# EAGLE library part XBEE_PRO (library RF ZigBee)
XBee , ZigBee transceiver Producted by XBee ; Digi-Key.Co
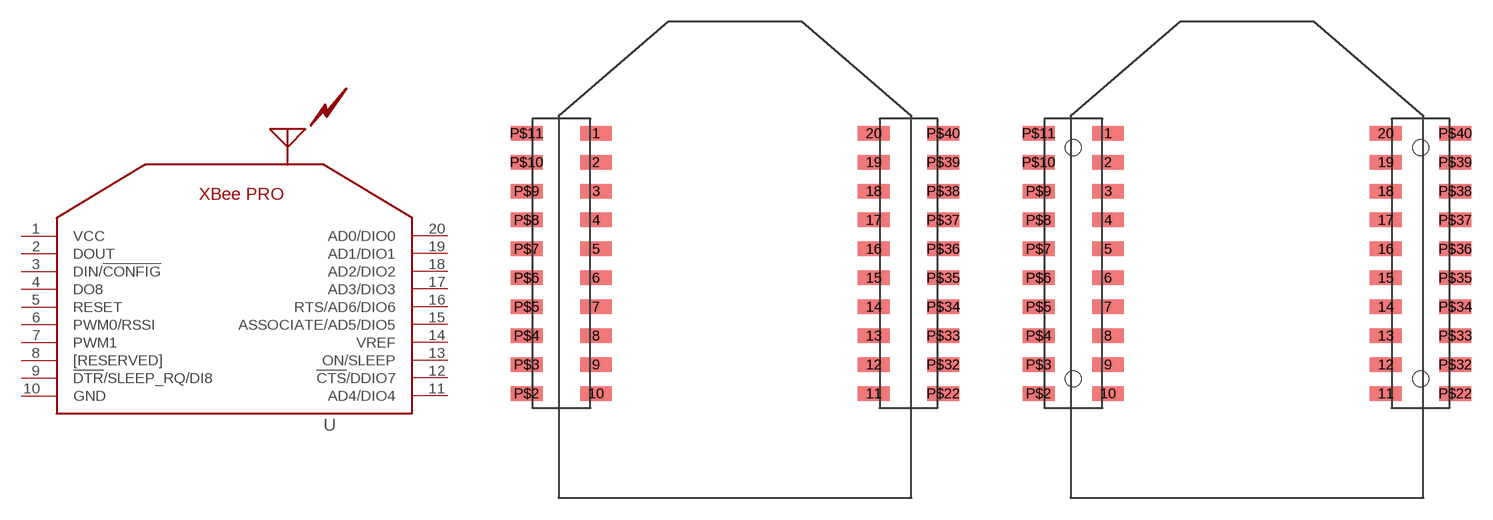
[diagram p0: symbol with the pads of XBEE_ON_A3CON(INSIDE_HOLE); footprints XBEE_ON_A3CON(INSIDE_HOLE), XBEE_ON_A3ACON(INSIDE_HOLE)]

Designator prefix U

## XBEE_PROA3-INSIDE_HOLE  [XBEE_ON_A3CON(INSIDE_HOLE)]
1  VCC
2  DOUT
3  DIN/!CONFIG
4  DO8
5  RESET
6  PWM0/RSSI
7  PWM1
8  [RESERVED]
9  !DTR!/SLEEP_RQ/DI8
10  GND
11  AD4/DIO4
12  !CTS!/DDIO7
13  ON/SLEEP
14  VREF
15  ASSOCIATE/AD5/DIO5
16  RTS/AD6/DIO6
17  AD3/DIO3
18  AD2/DIO2
19  AD1/DIO1
20  AD0/DIO0

## XBEE_PROA3A-INSIDE_HOLE  [XBEE_ON_A3ACON(INSIDE_HOLE)]
Pads as for XBEE_ON_A3CON(INSIDE_HOLE)

## XBEE_PRONPPN101BFLD-RC  [XBEE_ON_NPPN101BFLD-RC]
Pads as for XBEE_ON_A3CON(INSIDE_HOLE)

## XBEE_PROXPPN101BFCN  [XBEE_ON_XPPN101BFCN-RC]
Pads as for XBEE_ON_A3CON(INSIDE_HOLE)

## XBEE_PRONPPN101BFLC  [XBEE_ON_NPPN101BFLC-RC]
Pads as for XBEE_ON_A3CON(INSIDE_HOLE)

## Footprint XBEE_ON_A3CON(INSIDE_HOLE) (pad centres in mm)
XBee Pro on A3 receptacle connector (use inside sockets) ***Attention!!*** connector has not positioning adjustment holes! ****************** Producted by A3A connector ; Hirose.Co (HRS) XBee ;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
smd 2.2 x 1: 1 -9.6,18; 2 -9.6,16; 3 -9.6,14; 4 -9.6,12; 5 -9.6,10; 6 -9.6,8; 7 -9.6,6; 8 -9.6,4; 9 -9.6,2; 10 -9.6,0; 11 9.6,0; 12 9.6,2; 13 9.6,4; 14 9.6,6; 15 9.6,8; 16 9.6,10; 17 9.6,12; 18 9.6,14; 19 9.6,16; 20 9.6,18; P$2 -14.4,0; P$3 -14.4,2; P$4 -14.4,4; P$5 -14.4,6; P$6 -14.4,8; P$7 -14.4,10; P$8 -14.4,12; P$9 -14.4,14; P$10 -14.4,16; P$11 -14.4,18; P$22 14.4,0; P$32 14.4,2; P$33 14.4,4; P$34 14.4,6; P$35 14.4,8; P$36 14.4,10; P$37 14.4,12; P$38 14.4,14; P$39 14.4,16; P$40 14.4,18

## Footprint XBEE_ON_A3ACON(INSIDE_HOLE) (pad centres in mm)
XBee Pro on A3A receptacle connector (use inside sockets) ***Attention!!*** connector has 2 holes to position adjustment. ****************** Producted by A3A connector ; Hirose.Co (HRS) XBee ;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
smd 2.2 x 1: 1 -9.6,18; 2 -9.6,16; 3 -9.6,14; 4 -9.6,12; 5 -9.6,10; 6 -9.6,8; 7 -9.6,6; 8 -9.6,4; 9 -9.6,2; 10 -9.6,0; 11 9.6,0; 12 9.6,2; 13 9.6,4; 14 9.6,6; 15 9.6,8; 16 9.6,10; 17 9.6,12; 18 9.6,14; 19 9.6,16; 20 9.6,18; P$2 -14.4,0; P$3 -14.4,2; P$4 -14.4,4; P$5 -14.4,6; P$6 -14.4,8; P$7 -14.4,10; P$8 -14.4,12; P$9 -14.4,14; P$10 -14.4,16; P$11 -14.4,18; P$22 14.4,0; P$32 14.4,2; P$33 14.4,4; P$34 14.4,6; P$35 14.4,8; P$36 14.4,10; P$37 14.4,12; P$38 14.4,14; P$39 14.4,16; P$40 14.4,18
hole 1.1 at -12,1
hole 1.1 at -12,17
hole 1.1 at 12,17
hole 1.1 at 12,1

## Footprint XBEE_ON_NPPN101BFLD-RC (pad centres in mm)
XBee Pro on NPPN101BFLD-RC receptacle connector (1*10) Producted by XBee ; Digi-Key.Co Store: NPPN101BFLD-RC connector : Digi-Key.Co http://dkc1.digikey.com/jp/digihome.html
smd 2.29 x 0.89: 1 -12.395,18; 2 -9.605,16; 3 -12.395,14; 4 -9.605,12; 5 -12.395,10; 6 -9.605,8; 7 -12.395,6; 8 -9.605,4; 9 -12.395,2; 10 -9.605,0; 11 12.395,0; 12 9.605,2; 13 12.395,4; 14 9.605,6; 15 12.395,8; 16 9.605,10; 17 12.395,12; 18 9.605,14; 19 12.395,16; 20 9.605,18

## Footprint XBEE_ON_XPPN101BFCN-RC (pad centres in mm)
XBee Pro on NPPN101BFLD-RC receptacle connector (1*10) Producted by XBee ; Digi-Key.Co Store: NPPN101BFLC-RC connector : Digi-Key.Co http://dkc1.digikey.com/jp/digihome.html
drill 0.9: 1 -11,18; 2 -11,16; 3 -11,14; 4 -11,12; 5 -11,10; 6 -11,8; 7 -11,6; 8 -11,4; 9 -11,2; 10 -11,0; 11 11,0; 12 11,2; 13 11,4; 14 11,6; 15 11,8; 16 11,10; 17 11,12; 18 11,14; 19 11,16; 20 11,18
